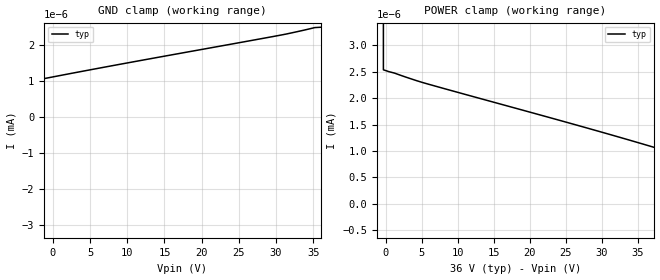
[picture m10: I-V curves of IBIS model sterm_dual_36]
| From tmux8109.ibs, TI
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| sterm_dual_36
[Model]   sterm_dual_36
Model_type   Terminator
|   typ   min   max
C_comp   2.533030e-12   NA   NA
[Voltage Range]   36   NA   NA
[Temperature Range]   27   NA   NA
[Power Clamp Reference]   36   NA   NA
[GND Clamp Reference]   0   NA   NA
[GND Clamp]
|   Voltage   I(typ)   I(min)   I(max)
-41V      -1.133A    NA         NA
-37.11V   -35.61mA   NA         NA
-36.33V   -3.132nA   NA         NA
-35.56V   -505.5pA   NA         NA
-30.89V   -313.9pA   NA         NA
-17.67V   352.5pA    NA         NA
-6V       874.7pA    NA         NA
7.222V    1.404nA    NA         NA
30.56V    2.284nA    NA         NA
35.22V    2.497nA    NA         NA
36V       2.506nA    NA         NA
[POWER Clamp]
|   Voltage   I(typ)   I(min)   I(max)
-5V       744mA      NA         NA
-1.111V   26.13mA    NA         NA
-333.3mV  2.538nA    NA         NA
5.111V    2.297nA    NA         NA
29.22V    1.387nA    NA         NA
42.44V    856pA      NA         NA
53.33V    368.5pA    NA         NA
67.33V    -334.5pA   NA         NA
72V       -522.1pA   NA         NA
